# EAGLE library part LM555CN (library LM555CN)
Single Timer
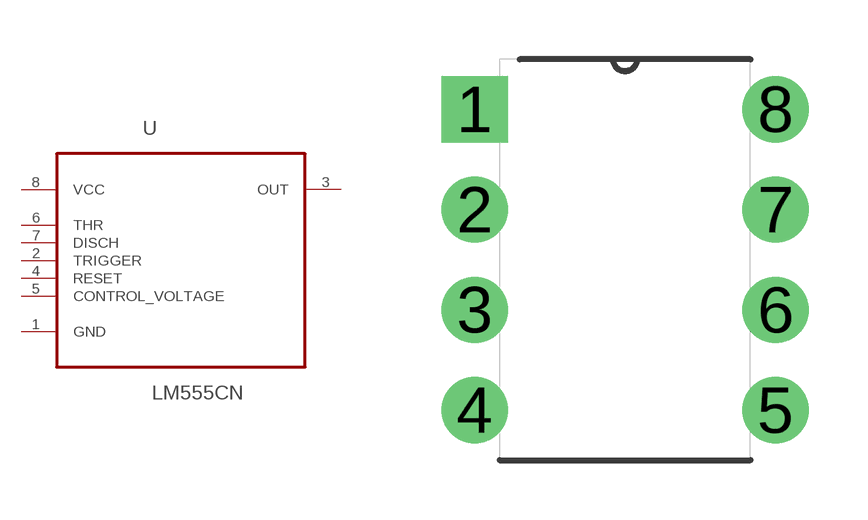
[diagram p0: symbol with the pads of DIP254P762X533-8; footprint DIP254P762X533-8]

Designator prefix U

## LM555CN (Availability: Unavailable; Description: Highly stable 555 timer for generating accurate time delays and oscillation 8-PDIP 0 to 70; MF: Texas Instruments; MP: LM555CN/NOPB; Package: DIP-8 Texas Instruments; Price: None)  [DIP254P762X533-8]
1  GND  pas
2  TRIGGER  in
3  OUT  out
4  RESET  in
5  CONTROL_VOLTAGE  in
6  THR  in
7  DISCH  in
8  VCC  pwr

## Footprint DIP254P762X533-8 (pad centres in mm)
drill 1.118 square: 1 -7.62,7.62
drill 1.118: 2 -7.62,5.08; 3 -7.62,2.54; 4 -7.62,0; 5 0,0; 6 0,2.54; 7 0,5.08; 8 0,7.62

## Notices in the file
This work is licensed under a Creative Commons Attribution-ShareAlike 4.0 International License (CC BY-SA) with Design Exception 1.0
